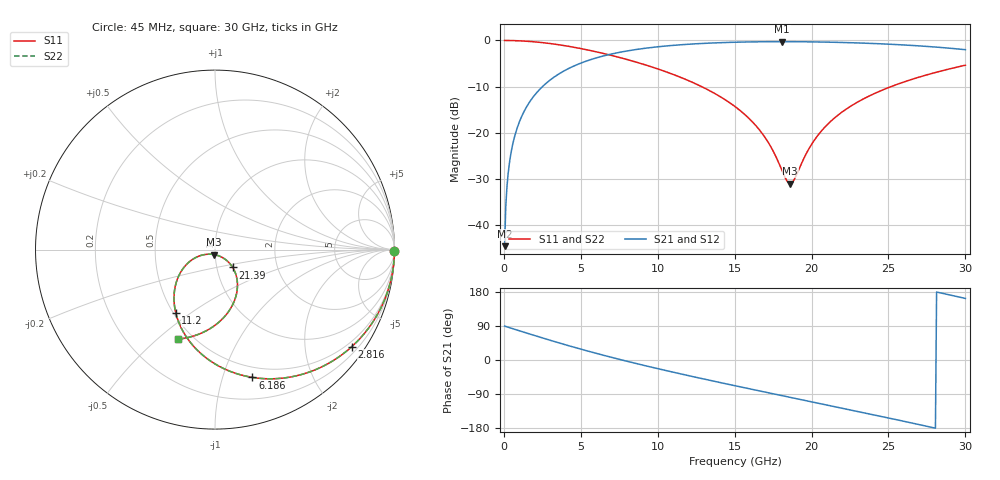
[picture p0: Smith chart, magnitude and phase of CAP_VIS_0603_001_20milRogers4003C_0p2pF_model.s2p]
! S-parameter model data by Modelithics Inc.  support@modelithics.com  813-866-6335  Tampa FL USA
! S-Parameter data specifications:
! Substrate: 20-mil Rogers 4003C, substrate thickness, H=0.508mm, Dielectric constant, Er=3.75
! PCB Mounting Pad Footprint: Pad width, PadW=0.90mm , Pad length, PadL=1.00mm , Pad gap, PadG (edge-to-edge)=1.00mm , Reference planes=3.0mm apart
! Created Wed Nov 18 13:15:44 2015
# hz S ma R 50
! 2 Port Network Data from SP1.SP block
! freq  magS11  angS11  magS21  angS21  magS12  angS12  magS22  angS22
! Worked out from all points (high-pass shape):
!   401 points, 45 MHz to 30 GHz, reference 50 ohm
!   highest |S21| = -0.26 dB at 18.09 GHz (marker M1); lowest = -44.5 dB at 45 MHz (marker M2)
!   |S21| within 3 dB of the highest: 6.578 GHz to end of sweep
!   lowest |S11| = -31.0 dB at 18.62 GHz (marker M3), VSWR 1.06, Z = 49.5 - j2.76 ohm
!   |S11| at or under -10 dB: 12.86 GHz to 25.16 GHz (12.3 GHz wide, 64.7 % of centre)
!   |S22| runs from -31.0 to 0.0 dB; largest |S21 - S12| = 0
!   S11 on the Smith chart (normalised r, x): 45 MHz: open; 2.816 GHz: 0.36, -3.10; 6.186 GHz: 0.40, -1.26; 11.2 GHz: 0.51, -0.44; 21.39 GHz: 1.19, -0.24; 30 GHz: 0.42, -0.59
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4.5e7  1 -0.6  0.005932 89.4  0.005932 89.4  1 -0.6
2.696625e8  0.9993 -3.4  0.03551 86.5  0.03551 86.5  0.9993 -3.4
3.4455e8  0.9989 -4.4  0.04535 85.5  0.04535 85.5  0.9989 -4.4
5.692125e8  0.9971 -7.3  0.07479 82.7  0.07479 82.7  0.9971 -7.3
7.93875e8  0.9943 -10.1  0.1041 79.8  0.1041 79.8  0.9943 -10.1
1.617638e9  0.9773 -20.6  0.2092 69.3  0.2092 69.3  0.9773 -20.6
2.815838e9  0.9343 -35.4  0.352 54.4  0.352 54.4  0.9343 -35.4
5.062462e9  0.8132 -61.5  0.5739 28.0  0.5739 28.0  0.8132 -61.5
6.185775e9  0.7419 -73.7  0.6604 15.6  0.6604 15.6  0.7419 -73.7
8.13285e9  0.6136 -93.5  0.7761 -4.7  0.7761 -4.7  0.6136 -93.5
1.007992e10  0.4869 -111.7  0.8567 -23.6  0.8567 -23.6  0.4869 -111.7
1.120324e10  0.4163 -121.6  0.8906 -34.0  0.8906 -34.0  0.4163 -121.6
1.50225e10  0.1925 -151.0  0.9569 -67.9  0.9569 -67.9  0.1925 -151.0
1.68198e10  0.09697 -157.9  0.9683 -83.3  0.9683 -83.3  0.09697 -157.9
1.809289e10  0.03861 -138.7  0.9704 -94.1  0.9704 -94.1  0.03861 -138.7
1.86171e10  0.02823 -99.3  0.97 -98.6  0.97 -98.6  0.02823 -99.3
1.891665e10  0.03223 -73.8  0.9694 -101.1  0.9694 -101.1  0.03223 -73.8
2.003996e10  0.07687 -43.7  0.9654 -110.6  0.9654 -110.6  0.07687 -43.7
2.138794e10  0.1399 -45.2  0.9565 -122.0  0.9565 -122.0  0.1399 -45.2
2.505742e10  0.3115 -70.3  0.9109 -153.5  0.9109 -153.5  0.3115 -70.3
2.745382e10  0.4225 -90.1  0.8632 -174.6  0.8632 -174.6  0.4225 -90.1
3e10  0.5394 -112.3  0.7946 162.4  0.7946 162.4  0.5394 -112.3
